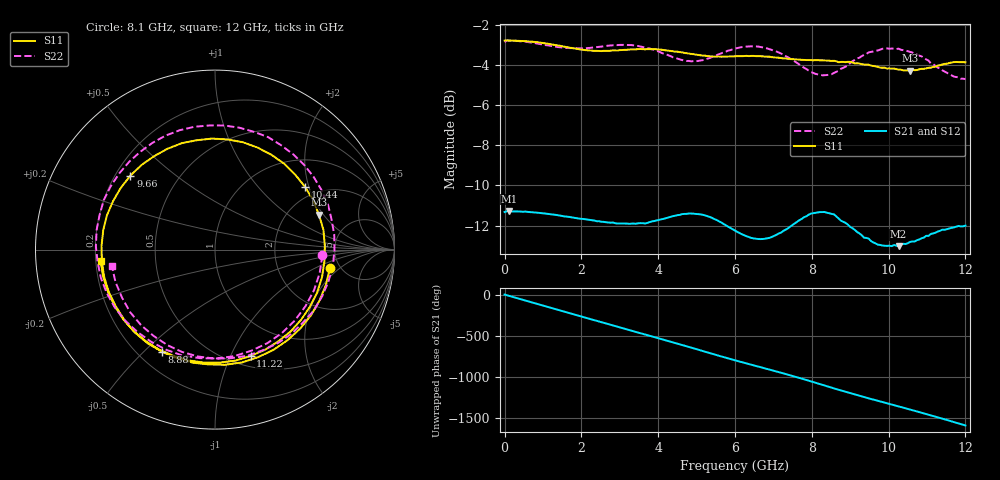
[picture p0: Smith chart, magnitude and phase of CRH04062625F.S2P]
!Agilent Technologies,E5071C,MY46109174,A.10.05
!Date: Wed Jun 26 07:19:23 2013
!Data & Calibration Information:
!Freq	S11:SOLT2(ON)	S21:SOLT2(ON)	S12:SOLT2(ON)	S22:SOLT2(ON)
!PortZ  Port1:50+j0  Port2:50+j0
!Above PortZ is port z conversion or system Z0 setting when saving the data.
!When reading, reference impedance value at option line is always used.
# Hz S dB R 50
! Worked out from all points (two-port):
!   201 points, 300 kHz to 12 GHz, reference 50 ohm
!   highest |S21| = -11.27 dB at 120.3 MHz (marker M1); lowest = -13.0 dB at 10.26 GHz (marker M2)
!   |S21| within 3 dB of the highest: start of sweep to end of sweep
!   lowest |S11| = -4.3 dB at 10.56 GHz (marker M3), VSWR 4.14, Z = 146 + j90.4 ohm
!   |S11| at or under -10 dB: nowhere
!   |S22| runs from -4.7 to -2.8 dB; largest |S21 - S12| = 0.0028
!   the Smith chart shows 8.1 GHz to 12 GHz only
!   S11 on the Smith chart (normalised r, x): 8.1 GHz: 4.13, -1.48; 8.88 GHz: 0.29, -0.57; 9.66 GHz: 0.26, +0.35; 10.44 GHz: 1.70, +1.89; 11.22 GHz: 0.61, -1.19; 12 GHz: 0.22, -0.05
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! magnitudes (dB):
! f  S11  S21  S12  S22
! 300 kHz  -2.8  -11.3  -11.3  -2.9
! 120.3 MHz  -2.8  -11.3  -11.3  -2.8
! 2.04 GHz  -3.2  -11.7  -11.7  -3.2
! 3.3 GHz  -3.2  -11.9  -11.9  -3.0
! 4.02 GHz  -3.2  -11.7  -11.7  -3.3
! 4.62 GHz  -3.4  -11.4  -11.4  -3.8
! 5.04 GHz  -3.5  -11.4  -11.4  -3.8
! 6 GHz  -3.6  -12.3  -12.2  -3.2
! 6.48 GHz  -3.5  -12.6  -12.6  -3.1
! 6.9 GHz  -3.6  -12.6  -12.6  -3.2
! 8.04 GHz  -3.8  -11.4  -11.4  -4.4
! 8.1 GHz  -3.8  -11.4  -11.4  -4.4
! 8.46 GHz  -3.8  -11.4  -11.4  -4.5
! 8.88 GHz  -3.9  -11.9  -11.9  -4.1
! 9.66 GHz  -4.1  -12.9  -12.9  -3.3
! 10.02 GHz  -4.2  -13.0  -13.0  -3.2
! 10.26 GHz  -4.2  -13.0  -13.0  -3.2
! 10.44 GHz  -4.3  -12.9  -12.9  -3.3
! 10.56 GHz  -4.3  -12.8  -12.8  -3.4
! 11.22 GHz  -4.1  -12.4  -12.3  -4.0
! 11.7 GHz  -3.9  -12.1  -12.1  -4.6
! 12 GHz  -3.9  -12.0  -12.0  -4.7
